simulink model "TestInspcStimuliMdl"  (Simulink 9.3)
settings: Solver=FixedStepDiscrete  StartTime=0.0  StopTime=10  FixedStep=Tstep  RelTol=1e-3
PreLoadFcn:
  | inspcStimuli.TestInspcStimuli_init();
InitFcn:
  | inspcStimuli.TestInspcStimuli_init();
StartFcn:
  | inspcStimuli.TestInspcStimuli_init();
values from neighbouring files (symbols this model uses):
  Tstep = 0.0001    [TestInspcStimuli_init.m]    (also in InspcCtrl_init.m; TestOrthOscObjO_init.m = 0.0005; stimuli_Smlk.m = 0.001; TestOrthOsc_init.m = 5e-05)
undefined symbols (not defined in the file or in its folder): T1, TI
libraries: libVishia_Inspc x4

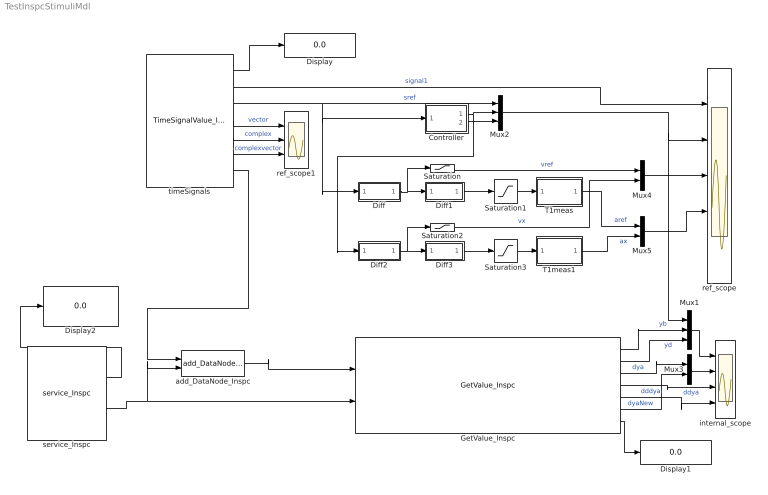
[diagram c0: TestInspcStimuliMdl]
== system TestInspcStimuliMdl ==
  Controller : Subsystem
  Diff : Subsystem
  Diff1 : Subsystem
  Diff2 : Subsystem
  Diff3 : Subsystem
  Display : Display
  Display1 : Display
  Display2 : Display
  GetValue_Inspc : libVishia_Inspc/GetValue_Inspc  Tstep=Tstep  path1='timeSignals.super.curr[1].yb[0]'  path2='timeSignals.super.curr[1].yd[0]'  path3='timeSignals.super.curr[1].dya[0]'  path4='timeSignals.super.curr[1].ddya[0]'  path5='timeSignals.super.curr[1].dddya[0]'  path6='timeSignals.super.curr[1].dyaNew[0]'
  Mux1 : Mux  Inputs=3
  Mux2 : Mux  Inputs=3
  Mux3 : Mux  Inputs=2
  Mux4 : Mux  Inputs=2
  Mux5 : Mux  Inputs=2
  Saturation : Saturate  UpperLimit=50  LowerLimit=-50
  Saturation1 : Saturate  UpperLimit=500  LowerLimit=-500
  Saturation2 : Saturate  UpperLimit=50  LowerLimit=-50
  Saturation3 : Saturate  UpperLimit=500  LowerLimit=-500
  T1meas : Subsystem
  T1meas1 : Subsystem
  add_DataNode_Inspc : libVishia_Inspc/add_DataNode_Inspc  name1Refl='timeSignals'  name2Refl=''
  internal_scope : Scope  NumInputPorts=4
  ref_scope : Scope  NumInputPorts=5
  ref_scope1 : Scope  NumInputPorts=3
  service_Inspc : libVishia_Inspc/service_Inspc  Tstep=Tstep  IpPort='UDP:0.0.0.0:60094'
  timeSignals : libVishia_Inspc/TimeSignalValue_Inspc  Description=|  Tstep=Tstep  filepath=timeSignalFilepath  nameRefl='timeSignals'  nrofStimuli=25  varDef=|
      | A combined stimuli and inspector function block.
      | Stimuli file path: file contains stimuli in form:
      |   %time:0: stimuli.namex = 5000.0, stimuli.namey = 50.0 -10; 
      | Name in reflection-tree: Name of this function block for stimuli and inspector access
      | name1..12: output type and name, base type is single always.
      | C2:namexy  A complex array of 2 elements
      | 6:namexy An array of 6 elements (max).
      | C:namexy  A 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
      | signal1:F;
      | sref:F*2;
      | vector:F*6;
      | complex:f;
      | complexvector:f*3;
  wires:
  timeSignals/1 -> Display/1
  timeSignals/3 -> Diff/1(In1), Controller/1(In1), Mux2/1  "sref"
  GetValue_Inspc/1 -> Mux1/2  "yb"
  add_DataNode_Inspc/1 -> GetValue_Inspc/1
  GetValue_Inspc/7 -> Display1/1
  GetValue_Inspc/2 -> Mux1/3  "yd"
  GetValue_Inspc/3 -> Mux3/1  "dya"
  Mux1/1 -> internal_scope/1
  GetValue_Inspc/5 -> internal_scope/4  "dddya"
  Controller/1(Out1) -> Diff2/1(In1), Mux2/2
  Mux2/1 -> Mux1/1, ref_scope/2
  GetValue_Inspc/4 -> internal_scope/3  "ddya"
  Mux3/1 -> internal_scope/2
  GetValue_Inspc/6 -> Mux3/2  "dyaNew"
  timeSignals/2 -> ref_scope/1  "signal1"
  Controller/2(Out2) -> Mux2/3
  Mux4/1 -> ref_scope/3
  Mux5/1 -> ref_scope/4
  service_Inspc/2 -> add_DataNode_Inspc/2, GetValue_Inspc/2
  timeSignals/7 -> add_DataNode_Inspc/1
  T1meas1/1(Out2) -> Mux5/2  "ax"
  Diff3/1(Out1) -> Saturation3/1
  Saturation2/1 -> Mux4/2  "vx"
  Diff2/1(Out1) -> Diff3/1(In1), Saturation2/1
  Saturation/1 -> Mux4/1  "vref"
  Saturation3/1 -> T1meas1/1(In2)
  T1meas/1(Out2) -> Mux5/1  "aref"
  Diff/1(Out1) -> Diff1/1(In1), Saturation/1
  Diff1/1(Out1) -> Saturation1/1
  Saturation1/1 -> T1meas/1(In2)
  timeSignals/6 -> ref_scope1/3  "complexvector"
  timeSignals/5 -> ref_scope1/2  "complex"
  timeSignals/4 -> ref_scope1/1  "vector"
  service_Inspc/1 -> Display2/1

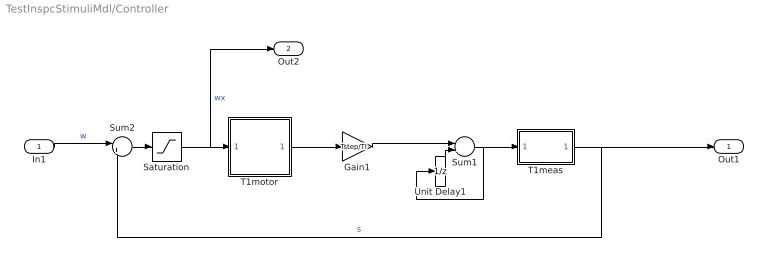
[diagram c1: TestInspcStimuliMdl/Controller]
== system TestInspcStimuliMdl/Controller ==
  In1 : Inport
  Gain1 : Gain  Gain=Tstep/TI
  Saturation : Saturate
  Sum1 : Sum  Inputs=|++
  Sum2 : Sum  Inputs=|+-
  T1meas : Subsystem
  T1motor : Subsystem
  Unit Delay1 : UnitDelay  SampleTime=-1  HasFrameUpgradeWarning=on
  Out1 : Outport
  Out2 : Outport  Port=2
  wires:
  T1meas/1(Out2) -> Sum2/2, Out1/1  "s"
  In1/1 -> Sum2/1  "w"
  Unit Delay1/1 -> Sum1/2
  Sum1/1 -> T1meas/1(In2), Unit Delay1/1
  Sum2/1 -> Saturation/1
  Gain1/1 -> Sum1/1
  T1motor/1(Out2) -> Gain1/1
  Saturation/1 -> Out2/1, T1motor/1(In2)  "wx"

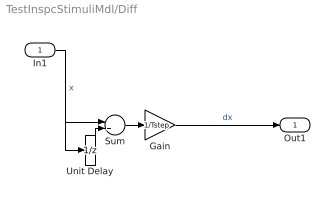
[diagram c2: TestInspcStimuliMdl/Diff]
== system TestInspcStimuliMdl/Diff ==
  In1 : Inport
  Gain : Gain  Gain=1/Tstep
  Sum : Sum  Inputs=|+-
  Unit Delay : UnitDelay  SampleTime=-1  HasFrameUpgradeWarning=on
  Out1 : Outport
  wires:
  Gain/1 -> Out1/1  "dx"
  In1/1 -> Unit Delay/1, Sum/1  "x"
  Unit Delay/1 -> Sum/2
  Sum/1 -> Gain/1

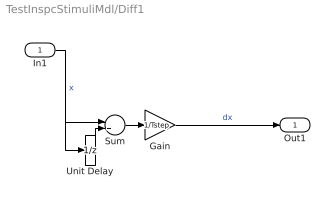
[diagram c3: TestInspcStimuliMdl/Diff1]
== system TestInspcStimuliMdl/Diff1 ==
  In1 : Inport
  Gain : Gain  Gain=1/Tstep
  Sum : Sum  Inputs=|+-
  Unit Delay : UnitDelay  SampleTime=-1  HasFrameUpgradeWarning=on
  Out1 : Outport
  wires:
  Gain/1 -> Out1/1  "dx"
  In1/1 -> Unit Delay/1, Sum/1  "x"
  Unit Delay/1 -> Sum/2
  Sum/1 -> Gain/1

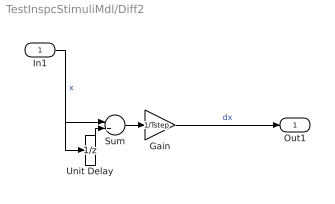
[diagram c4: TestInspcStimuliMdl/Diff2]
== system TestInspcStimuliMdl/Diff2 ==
  In1 : Inport
  Gain : Gain  Gain=1/Tstep
  Sum : Sum  Inputs=|+-
  Unit Delay : UnitDelay  SampleTime=-1  HasFrameUpgradeWarning=on
  Out1 : Outport
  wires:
  Gain/1 -> Out1/1  "dx"
  In1/1 -> Unit Delay/1, Sum/1  "x"
  Unit Delay/1 -> Sum/2
  Sum/1 -> Gain/1

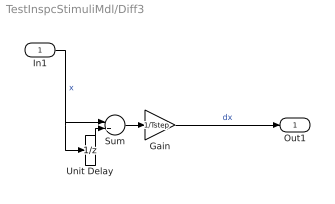
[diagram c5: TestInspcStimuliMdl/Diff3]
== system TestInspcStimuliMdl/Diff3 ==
  In1 : Inport
  Gain : Gain  Gain=1/Tstep
  Sum : Sum  Inputs=|+-
  Unit Delay : UnitDelay  SampleTime=-1  HasFrameUpgradeWarning=on
  Out1 : Outport
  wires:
  Gain/1 -> Out1/1  "dx"
  In1/1 -> Unit Delay/1, Sum/1  "x"
  Unit Delay/1 -> Sum/2
  Sum/1 -> Gain/1

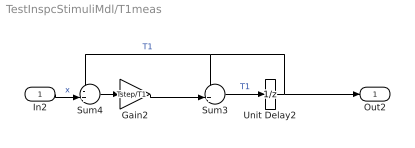
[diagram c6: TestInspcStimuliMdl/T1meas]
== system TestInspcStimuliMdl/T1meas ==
  In2 : Inport
  Gain2 : Gain  Gain=Tstep/T1
  Sum3 : Sum  Inputs=++|
  Sum4 : Sum  Inputs=-+|
  Unit Delay2 : UnitDelay  SampleTime=-1  HasFrameUpgradeWarning=on
  Out2 : Outport
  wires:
  Sum4/1 -> Gain2/1
  In2/1 -> Sum4/2  "x"
  Sum3/1 -> Unit Delay2/1  "T1"
  Gain2/1 -> Sum3/2
  Unit Delay2/1 -> Sum4/1, Sum3/1, Out2/1  "T1"

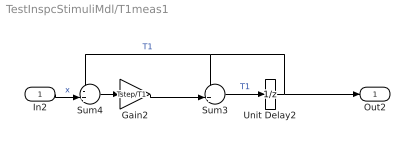
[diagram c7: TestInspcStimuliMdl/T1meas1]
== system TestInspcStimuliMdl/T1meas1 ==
  In2 : Inport
  Gain2 : Gain  Gain=Tstep/T1
  Sum3 : Sum  Inputs=++|
  Sum4 : Sum  Inputs=-+|
  Unit Delay2 : UnitDelay  SampleTime=-1  HasFrameUpgradeWarning=on
  Out2 : Outport
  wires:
  Sum4/1 -> Gain2/1
  In2/1 -> Sum4/2  "x"
  Sum3/1 -> Unit Delay2/1  "T1"
  Gain2/1 -> Sum3/2
  Unit Delay2/1 -> Sum4/1, Sum3/1, Out2/1  "T1"

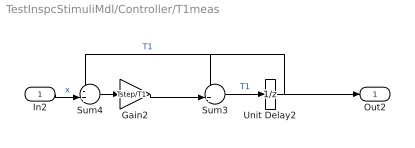
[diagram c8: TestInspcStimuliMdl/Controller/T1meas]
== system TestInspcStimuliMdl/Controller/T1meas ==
  In2 : Inport
  Gain2 : Gain  Gain=Tstep/T1
  Sum3 : Sum  Inputs=++|
  Sum4 : Sum  Inputs=-+|
  Unit Delay2 : UnitDelay  SampleTime=-1  HasFrameUpgradeWarning=on
  Out2 : Outport
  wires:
  Sum4/1 -> Gain2/1
  In2/1 -> Sum4/2  "x"
  Sum3/1 -> Unit Delay2/1  "T1"
  Gain2/1 -> Sum3/2
  Unit Delay2/1 -> Sum4/1, Sum3/1, Out2/1  "T1"

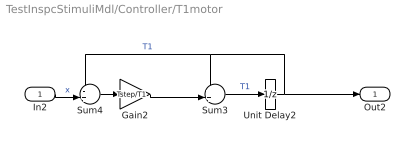
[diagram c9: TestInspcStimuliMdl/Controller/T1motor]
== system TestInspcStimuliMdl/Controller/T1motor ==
  In2 : Inport
  Gain2 : Gain  Gain=Tstep/T1
  Sum3 : Sum  Inputs=++|
  Sum4 : Sum  Inputs=-+|
  Unit Delay2 : UnitDelay  SampleTime=-1  HasFrameUpgradeWarning=on
  Out2 : Outport
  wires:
  Sum4/1 -> Gain2/1
  In2/1 -> Sum4/2  "x"
  Sum3/1 -> Unit Delay2/1  "T1"
  Gain2/1 -> Sum3/2
  Unit Delay2/1 -> Sum4/1, Sum3/1, Out2/1  "T1"
